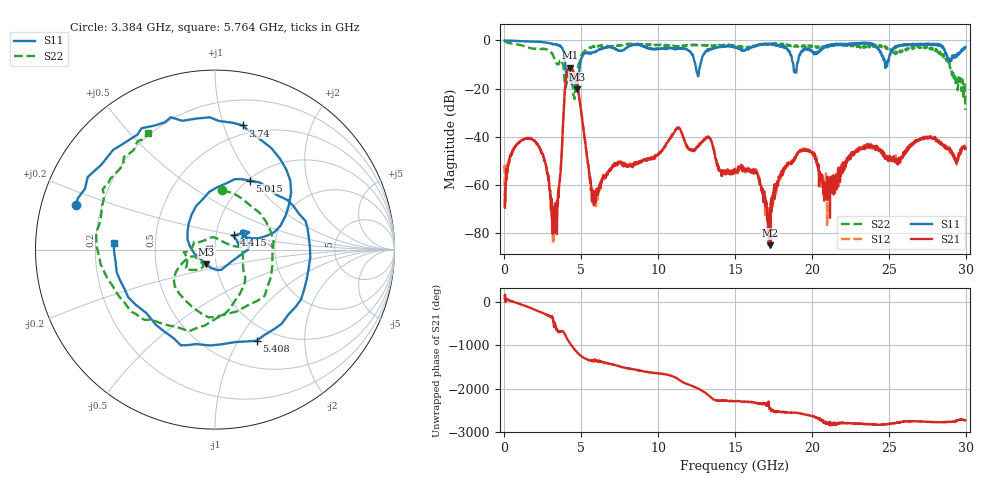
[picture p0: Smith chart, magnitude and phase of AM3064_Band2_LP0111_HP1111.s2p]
# Hz S DB R 50.0
!freq dBS11 angS11 dBS21 angS21 dBS12 angS12 dBS22 angS22
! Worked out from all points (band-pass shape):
!   1600 points, 10 MHz to 29.98 GHz, reference 50 ohm
!   highest |S21| = -11.30 dB at 4.246 GHz (marker M1); lowest = -85.1 dB at 17.29 GHz (marker M2)
!   |S21| within 3 dB of the highest: 4.035 GHz to 4.565 GHz (529.7 MHz wide, 12.3 % of centre)
!   lowest |S11| = -20.4 dB at 4.733 GHz (marker M3), VSWR 1.21, Z = 44.7 - j7.4 ohm
!   |S11| at or under -10 dB: 3.957 GHz to 4.917 GHz (959.8 MHz wide, 21.6 % of centre); 12.42 GHz to 12.75 GHz (331.2 MHz wide, 2.63 % of centre); 18.79 GHz to 19.03 GHz (243.1 MHz wide, 1.29 % of centre)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
!   |S22| runs from -28.9 to -0.2 dB; largest |S21 - S12| = 0.0087
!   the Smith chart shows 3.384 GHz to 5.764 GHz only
!   S11 on the Smith chart (normalised r, x): 3.384 GHz: 0.10, +0.16; 3.74 GHz: 0.42, +1.16; 4.415 GHz: 1.22, +0.20; 5.015 GHz: 1.02, +0.97; 5.408 GHz: 0.81, -1.20; 5.764 GHz: 0.28, +0.03
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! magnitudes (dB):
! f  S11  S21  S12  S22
! 10 MHz  -0.1  -66.2  -51.6  -0.2
! 572.3 MHz  -0.2  -45.4  -45.8  -1.4
! 1.734 GHz  -0.5  -40.9  -40.7  -3.3
! 3.384 GHz  -1.8  -78.8  -70.6  -9.6
! 3.74 GHz  -3.0  -44.9  -44.1  -8.8
! 4.246 GHz  -15.8  -11.3  -11.4  -15.7
! 4.415 GHz  -17.5  -12.2  -12.0  -18.1
! 4.733 GHz  -20.4  -18.8  -18.7  -12.8
! 5.015 GHz  -7.3  -30.8  -30.6  -6.3
! 5.408 GHz  -5.1  -49.6  -50.1  -3.5
! 5.764 GHz  -4.9  -66.0  -63.8  -2.5
! 10 GHz  -3.6  -46.9  -47.6  -2.0
! 11.31 GHz  -3.0  -36.5  -36.3  -2.6
! 15 GHz  -2.6  -54.6  -55.2  -2.0
! 16.34 GHz  -2.4  -54.6  -53.7  -2.5
! 17.29 GHz  -1.7  -85.1  -72.2  -1.4
! 18.3 GHz  -2.8  -52.5  -52.6  -2.2
! 19.99 GHz  -4.3  -46.6  -46.4  -2.2
! 21.02 GHz  -1.9  -57.4  -64.3  -2.6
! 25 GHz  -8.1  -48.8  -48.7  -3.1
! 28.31 GHz  -2.2  -42.4  -42.8  -4.7
! 29.98 GHz  -2.7  -44.6  -45.2  -28.9
